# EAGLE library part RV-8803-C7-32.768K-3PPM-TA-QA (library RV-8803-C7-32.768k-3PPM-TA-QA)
RV-8803-C7 8-Terminal Ceramic Leadless Chip Carrier [LCC8] Source: Datasheet
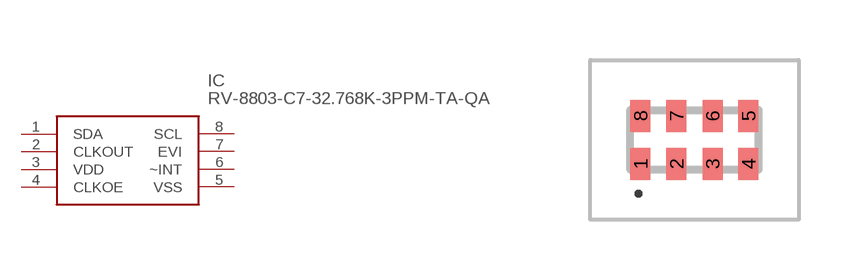
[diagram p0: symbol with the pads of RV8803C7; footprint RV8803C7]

Designator prefix IC

## RV-8803-C7-32.768K-3PPM-TA-QA (Description: RV-8803-C7 8-Terminal Ceramic Leadless Chip Carrier [LCC8]; Height: 0.8mm; Manufacturer_Name: Micro Crystal AG; Manufacturer_Part_Number: RV-8803-C7-32.768k-3PPM-TA-QA; Mouser_Part_Number: 428-203035-MG01; Mouser_Price-Stock: https://www.mouser.co.uk/ProductDetail/Micro-Crystal/RV-8803-C7-32.768k-3PPM-TA-QA?qs=7bTaA%2FLYtSb5zZOilbtzxw%3D%3D)  [RV8803C7]
1  SDA
2  CLKOUT
3  VDD
4  CLKOE
5  VSS
6  ~INT
7  EVI
8  SCL

## Footprint RV8803C7 (pad centres in mm)
SON-8
smd 0.5 x 0.8: 1 -1.35,-0.6; 2 -0.45,-0.6; 3 0.45,-0.6; 4 1.35,-0.6; 5 1.35,0.6; 6 0.45,0.6; 7 -0.45,0.6; 8 -1.35,0.6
